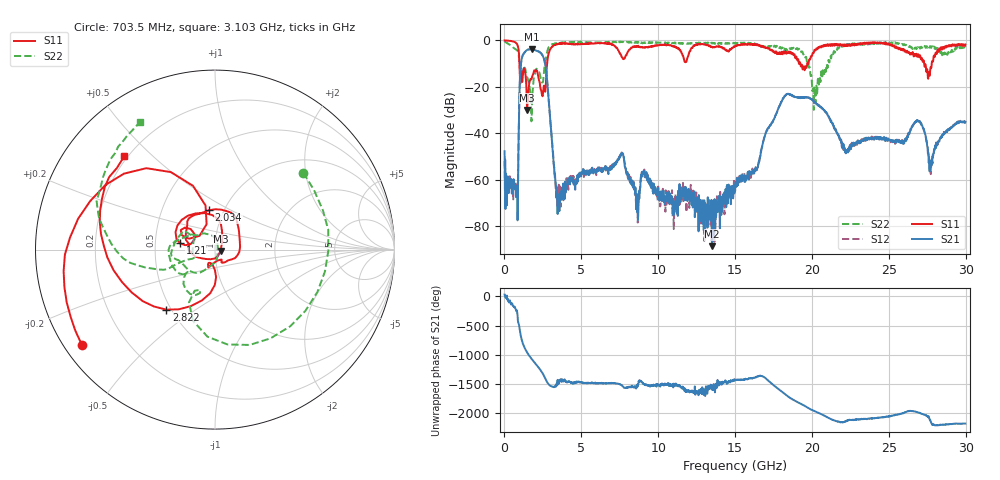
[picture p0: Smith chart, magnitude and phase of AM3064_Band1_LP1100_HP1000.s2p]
# Hz S DB R 50.0
!freq dBS11 angS11 dBS21 angS21 dBS12 angS12 dBS22 angS22
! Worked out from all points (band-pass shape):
!   1600 points, 10 MHz to 29.98 GHz, reference 50 ohm
!   highest |S21| = -3.80 dB at 1.791 GHz (marker M1); lowest = -88.5 dB at 13.51 GHz (marker M2)
!   |S21| within 3 dB of the highest: 1.167 GHz to 2.502 GHz (1.335 GHz wide, 72.8 % of centre)
!   lowest |S11| = -30.0 dB at 1.472 GHz (marker M3), VSWR 1.07, Z = 53.2 - j0.762 ohm
!   |S11| at or under -10 dB: 974 MHz to 2.775 GHz (1.801 GHz wide, 96.1 % of centre); 19.24 GHz to 19.69 GHz (448.8 MHz wide, 2.31 % of centre); 27.3 GHz to 27.79 GHz (494.2 MHz wide, 1.79 % of centre)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
!   |S22| runs from -34.8 to -0.5 dB; largest |S21 - S12| = 0.0089
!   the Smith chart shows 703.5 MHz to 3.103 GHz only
!   S11 on the Smith chart (normalised r, x): 703.5 MHz: 0.05, -0.32; 1.21 GHz: 0.67, +0.05; 2.034 GHz: 0.85, +0.39; 2.822 GHz: 0.47, -0.39; 3.103 GHz: 0.19, +0.41
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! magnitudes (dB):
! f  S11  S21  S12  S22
! 10 MHz  0.0  -47.7  -51.9  -0.5
! 703.5 MHz  -0.8  -62.4  -62.9  -3.7
! 1.21 GHz  -14.0  -6.2  -6.1  -12.9
! 1.472 GHz  -30.0  -4.2  -4.1  -15.9
! 1.791 GHz  -15.8  -3.8  -3.8  -27.8
! 2.034 GHz  -13.1  -4.3  -4.3  -12.9
! 2.822 GHz  -7.3  -20.9  -20.9  -3.9
! 3.103 GHz  -2.8  -44.2  -44.2  -1.7
! 3.515 GHz  -1.5  -70.0  -65.4  -1.1
! 5.015 GHz  -1.6  -57.2  -57.9  -0.6
! 7.62 GHz  -7.1  -48.8  -48.2  -0.7
! 8.632 GHz  -2.8  -70.5  -73.6  -1.0
! 10 GHz  -2.1  -63.5  -62.9  -1.0
! 13.51 GHz  -2.8  -88.5  -74.3  -1.1
! 15 GHz  -2.7  -63.2  -64.8  -1.3
! 18.25 GHz  -5.1  -23.8  -23.9  -4.3
! 19.99 GHz  -6.8  -25.5  -25.5  -17.4
! 22.2 GHz  -1.8  -48.6  -47.7  -2.3
! 25 GHz  -1.3  -42.6  -42.9  -1.2
! 26.94 GHz  -6.4  -34.8  -34.7  -3.3
! 27.77 GHz  -11.6  -53.9  -51.4  -3.1
! 29.98 GHz  -1.8  -35.1  -34.8  -2.9
